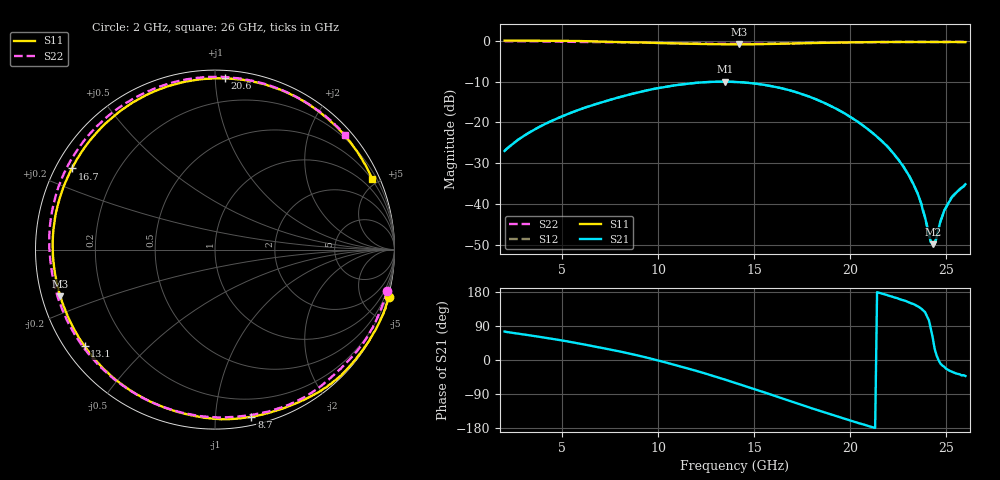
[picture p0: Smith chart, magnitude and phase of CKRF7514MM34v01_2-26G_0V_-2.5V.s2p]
! CHUO DENSHI KOGYO Co.,Ltd.
! 30. May 2016
! CKRF7514MM34
! N-channel HJ-FET
! Vds = 0 V Vgs = -2.5 V
# Hz S  MA  R 50
!  f  S11  S21  S12  S22
!  Hz  MAG  ANG  MAG  ANG  MAG  ANG  MAG  ANG
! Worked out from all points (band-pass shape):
!   241 points, 2 GHz to 26 GHz, reference 50 ohm
!   highest |S21| = -10.03 dB at 13.5 GHz (marker M1); lowest = -49.8 dB at 24.3 GHz (marker M2)
!   |S21| within 3 dB of the highest: 8.63 GHz to 17.47 GHz (8.836 GHz wide, 67.7 % of centre)
!   lowest |S11| = -0.9 dB at 14.2 GHz (marker M3), VSWR 18.92, Z = 2.7 - j7.37 ohm
!   |S11| at or under -10 dB: nowhere
!   |S22| runs from -0.8 to -0.1 dB; largest |S21 - S12| = 0.00065
!   S11 on the Smith chart (normalised r, x): 2 GHz: -0.11, -7.43; 8.7 GHz: 0.06, -1.24; 13.1 GHz: 0.06, -0.33; 16.7 GHz: 0.05, +0.26; 20.6 GHz: 0.05, +1.06; 26 GHz: 0.47, +4.65
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2e9  1.004 -15.3  0.04482 75.0  0.04475 74.9  0.9866 -13.4
3.5e9  0.9994 -27.1  0.08053 63.5  0.08061 63.6  0.9807 -24.1
6e9  0.9882 -49.0  0.1467 42.3  0.1462 42.4  0.9632 -44.2
8.7e9  0.9531 -77.7  0.2252 14.8  0.225 14.8  0.9502 -71.1
1e10  0.9365 -94.7  0.2628 -1.2  0.2628 -1.3  0.9368 -86.1
1.16e10  0.917 -118.3  0.2985 -23.0  0.2987 -23.0  0.9236 -106.7
1.31e10  0.904 -143.4  0.3147 -45.7  0.3146 -45.7  0.9148 -128.0
1.35e10  0.9019 -150.5  0.3152 -52.1  0.3152 -52.0  0.9135 -134.0
1.4e10  0.9001 -159.6  0.3124 -60.2  0.3124 -60.1  0.9129 -141.6
1.42e10  0.8996 -163.2  0.311 -63.4  0.3108 -63.4  0.9132 -144.6
1.55e10  0.9071 172.6  0.2886 -85.0  0.2882 -85.0  0.9152 -164.7
1.67e10  0.9169 150.4  0.2525 -105.4  0.2525 -105.3  0.9255 176.4
1.8e10  0.933 127.4  0.201 -127.5  0.2006 -127.4  0.9408 155.2
1.93e10  0.9473 106.0  0.1458 -148.5  0.1456 -148.4  0.9516 134.1
2.06e10  0.956 86.6  0.09413 -168.7  0.09439 -168.7  0.9579 113.6
2.2e10  0.9628 67.7  0.04891 169.7  0.049 170.2  0.9632 92.5
2.34e10  0.9625 51.0  0.01542 145.0  0.01553 146.4  0.9637 72.9
2.43e10  0.9624 41.0  0.003221 58.6  0.003063 57.8  0.9637 61.1
2.44e10  0.9625 40.0  0.003248 29.2  0.003318 29.6  0.9637 60.0
2.49e10  0.962 34.8  0.008392 -18.0  0.008362 -19.8  0.9638 53.9
2.52e10  0.9613 31.7  0.01106 -29.0  0.01136 -28.1  0.9654 50.3
2.6e10  0.9593 24.1  0.01753 -42.1  0.01737 -41.8  0.9664 41.4
